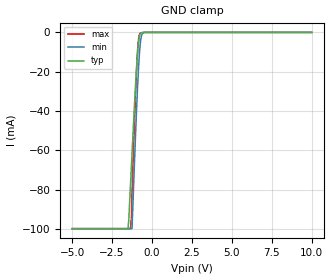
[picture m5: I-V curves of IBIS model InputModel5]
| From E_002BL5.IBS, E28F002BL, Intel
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|*********************Input Model 5*********************************
[Model]   InputModel5
Model_type   Input
|   Model for WE# pin.
Vinl = 0.8V
Vinh = 2.0V
|Variable   Typ   Min   Max
C_comp   5.61p   NA   7.6p
[Voltage Range]   5.0V   4.5V   5.5V
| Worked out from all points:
|   GND clamp passes 1 mA (typ) near -0.75 V on its own axis
[GND_clamp]
|Voltage  I(typ)   I(min)   I(max)
-5V       -99.85mA   -99.85mA   -99.85mA
-1.5V     -99.85mA   -99.85mA   -99.85mA
-1.35V    -78.19mA   -99.85mA   -99.85mA
-1.3V     -69.95mA   -99.85mA   -95.52mA
-1.25V    -61.7mA    -99.85mA   -82.78mA
-1.1V     -37.45mA   -66.88mA   -46.7mA
-950mV    -15.91mA   -36.25mA   -16.07mA
-850mV    -5.765mA   -19.23mA   -3.761mA
-750mV    -1.018mA   -6.959mA   -470.1uA
-650mV    -205.8uA   -1.5mA     -137.6uA
-500mV    -27.27uA   0A         0A
10V       0A         0A         0A
[Power_clamp]
| Input buffer circuits of this product do not intrinsically
| require a [Power_clamp] definition.  This zero current
| [Power_clamp] table is provided for the compatibility with
| some IBIS parsers.
|Voltage  I(typ)   I(min)   I(max)
-5V       0A         0A         0A
0V        0A         0A         0A
5V        0A         0A         0A
10V       0A         0A         0A
